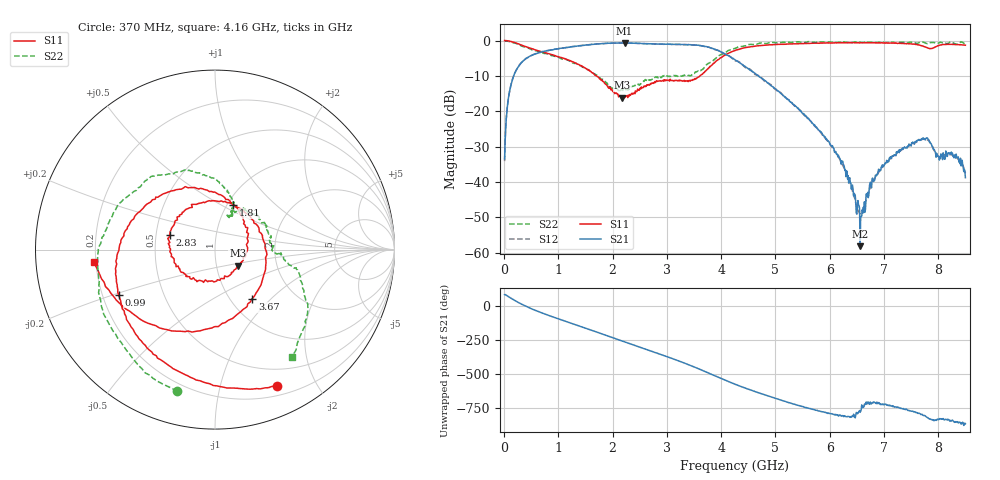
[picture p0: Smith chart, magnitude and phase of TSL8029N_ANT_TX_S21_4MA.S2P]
!Agilent Technologies,E5071C,MY46523237,B.13.01
!Date: Wed Oct 18 10:59:52 2023
!Data & Calibration Information:
!Freq	S11:SOLT2(ON)	S21:SOLT2(ON)	S12:SOLT2(ON)	S22:SOLT2(ON)
!PortZ  Port1:50+j0  Port2:50+j0
!Above PortZ is port z conversion or system Z0 setting when saving the data.
!When reading, reference impedance value at option line is always used.
# Hz S dB R 50
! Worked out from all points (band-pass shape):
!   850 points, 10 MHz to 8.5 GHz, reference 50 ohm
!   highest |S21| = -0.66 dB at 2.22 GHz (marker M1); lowest = -58.1 dB at 6.56 GHz (marker M2)
!   |S21| within 3 dB of the highest: 605.2 MHz to 4.056 GHz (3.451 GHz wide, 148 % of centre)
!   lowest |S11| = -16.2 dB at 2.18 GHz (marker M3), VSWR 1.37, Z = 63.4 - j11.6 ohm
!   |S11| at or under -10 dB: 1.706 GHz to 3.61 GHz (1.903 GHz wide, 71.6 % of centre)
!   |S22| runs from -14.2 to 0.0 dB; largest |S21 - S12| = 0.02
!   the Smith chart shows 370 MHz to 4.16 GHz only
!   S11 on the Smith chart (normalised r, x): 370 MHz: 0.30, -1.51; 990 MHz: 0.27, -0.21; 1.81 GHz: 1.07, +0.57; 2.83 GHz: 0.59, +0.10; 3.67 GHz: 1.25, -0.78; 4.16 GHz: 0.19, -0.05
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1e7  -0.02 -1.9  -33.48 83.8  -34.09 87.4  0.02 -3.0
1.3e8  -0.31 -25.1  -12.37 57.0  -12.34 56.4  -0.46 -40.9
3.7e8  -1.55 -65.7  -5.54 4.5  -5.49 4.5  -1.75 -104.9
6.2e8  -2.87 -102.2  -3.54 -38.8  -3.56 -38.7  -3.01 -153.4
9.9e8  -4.54 -154.9  -2.38 -92.8  -2.34 -92.8  -4.68 152.2
1.43e9  -7.11 138.4  -1.45 -153.4  -1.38 -153.4  -7.34 101.0
1.81e9  -11.40 68.0  -0.87 153.6  -0.87 153.9  -10.93 69.0
2.18e9  -16.16 -35.1  -0.67 101.4  -0.70 101.5  -13.95 68.5
2.22e9  -15.95 -51.3  -0.66 95.8  -0.70 95.9  -14.18 69.0
2.83e9  -11.52 162.6  -1.02 11.0  -1.00 10.7  -10.32 38.0
2.84e9  -11.47 159.5  -0.98 9.5  -0.99 9.2  -10.55 38.3
3.34e9  -11.51 49.8  -1.14 -63.2  -1.15 -63.5  -9.72 3.2
3.67e9  -9.28 -52.9  -1.59 -117.3  -1.61 -117.1  -8.04 -9.1
4.16e9  -3.42 -174.2  -4.56 159.0  -4.49 159.8  -2.65 -54.5
4.26e9  -2.79 165.8  -5.52 143.1  -5.74 143.3  -2.22 -66.2
4.78e9  -1.32 70.8  -11.09 68.3  -11.21 70.2  -0.80 -119.2
5.21e9  -0.99 -2.0  -16.53 12.9  -16.39 12.9  -0.41 -158.5
5.67e9  -0.78 -70.0  -23.18 -40.6  -23.24 -38.3  -0.48 163.5
6.56e9  -0.68 -170.3  -58.14 -63.6  -49.06 -46.7  -0.48 89.6
7.09e9  -0.74 135.1  -34.14 -11.0  -33.82 -12.7  -0.50 43.1
7.62e9  -1.18 77.5  -28.19 -66.1  -28.61 -69.1  -0.77 -5.3
8.5e9  -1.33 -21.2  -38.77 -148.2  -37.45 -148.8  -1.01 -89.1
